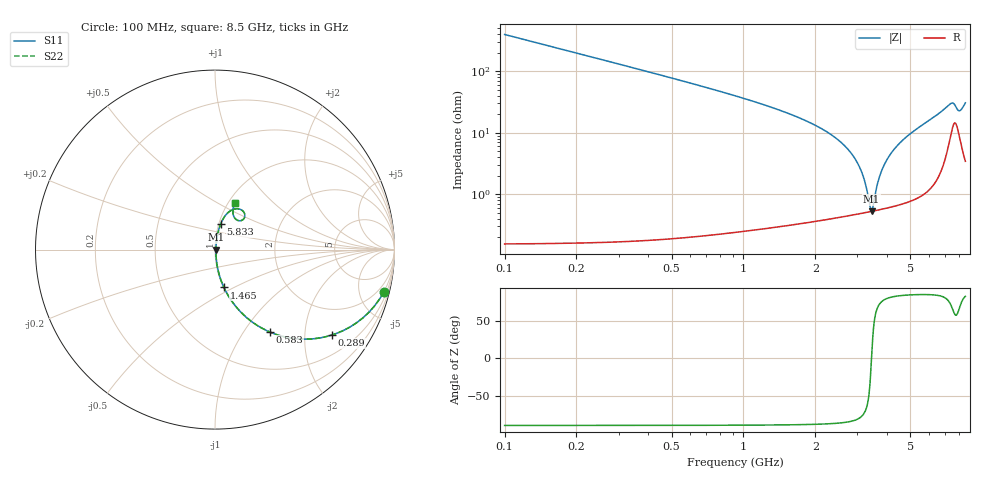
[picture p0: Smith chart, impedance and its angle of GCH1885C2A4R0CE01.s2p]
!Murata Part Number: GCH1885C2A4R0CE01
!These Parameters are Measured in Series Mode Connection
!Data Generated on Jun 19, 2026
!  o--ll--o
!Port1  Port2
!  o------o
!Operation Temp=25[degC], DC Bias Voltage=0[V]
!Freq. Start=100[MHz] Stop=9[GHz] 401[Steps]
# Hz S RI R 50
!Freq.(Hz) S11(Real) S11(Imag) S21(Real) S21(Imag) S12(Real) S12(Imag) S22(Real) S22(Imag)
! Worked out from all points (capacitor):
!   401 points, 100 MHz to 8.5 GHz, reference 50 ohm
!   read as one part in series: C = 4 pF near 142 MHz
!   lowest |Z| = 526 mohm at 3.439 GHz (marker M1)
!   series resonance near 3.438 GHz, so ESL is about 540 pH
!   S11 on the Smith chart (normalised r, x): 100 MHz: 1.00, -7.95; 289 MHz: 1.00, -2.73; 583 MHz: 1.00, -1.33; 1.465 GHz: 1.01, -0.45; 5.833 GHz: 1.02, +0.30; 8.5 GHz: 1.07, +0.61
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1e8  0.9404 -0.2365  0.0596 0.2365  0.0596 0.2365  0.9404 -0.2365
2.89e8  0.6512 -0.476  0.3488 0.476  0.3488 0.476  0.6512 -0.476
5.83e8  0.3057 -0.4592  0.6943 0.4592  0.6943 0.4592  0.3057 -0.4592
9.19e8  0.1406 -0.3447  0.8594 0.3447  0.8594 0.3447  0.1406 -0.3447
1.465e9  0.0498 -0.2109  0.9502 0.2109  0.9502 0.2109  0.0498 -0.2109
1.507e9  0.0463 -0.2032  0.9537 0.2032  0.9537 0.2032  0.0463 -0.2032
2.41e9  0.0111 -0.0835  0.9889 0.0835  0.9889 0.0835  0.0111 -0.0835
2.914e9  0.00613 -0.0387  0.9939 0.0387  0.9939 0.0387  0.00613 -0.0387
3.166e9  0.00529 -0.0193  0.9947 0.0193  0.9947 0.0193  0.00529 -0.0193
3.397e9  0.00519 -0.00282  0.9948 0.00282  0.9948 0.00282  0.00519 -0.00282
3.439e9  0.00524 6.69e-05  0.9948 -6.69e-05  0.9948 -6.69e-05  0.00524 6.69e-05
3.649e9  0.00569 0.0141  0.9943 -0.0141  0.9943 -0.0141  0.00569 0.0141
3.775e9  0.00614 0.0222  0.9939 -0.0222  0.9939 -0.0222  0.00614 0.0222
4.006e9  0.00729 0.0365  0.9927 -0.0365  0.9927 -0.0365  0.00729 0.0365
4.3e9  0.00932 0.0541  0.9907 -0.0541  0.9907 -0.0541  0.00932 0.0541
4.867e9  0.0149 0.0866  0.9851 -0.0866  0.9851 -0.0866  0.0149 0.0866
5.707e9  0.0285 0.1345  0.9715 -0.1345  0.9715 -0.1345  0.0285 0.1345
5.833e9  0.0314 0.1419  0.9686 -0.1419  0.9686 -0.1419  0.0314 0.1419
7.114e9  0.1017 0.2239  0.8983 -0.2239  0.8983 -0.2239  0.1017 0.2239
7.492e9  0.1582 0.2119  0.8418 -0.2119  0.8418 -0.2119  0.1582 0.2119
7.996e9  0.1159 0.1692  0.8841 -0.1692  0.8841 -0.1692  0.1159 0.1692
8.5e9  0.1106 0.2623  0.8894 -0.2623  0.8894 -0.2623  0.1106 0.2623
